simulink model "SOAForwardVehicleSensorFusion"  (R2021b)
settings: Solver=FixedStepAuto  StartTime=0.0  StopTime=scenario.StopTime  RelTol=1e-3

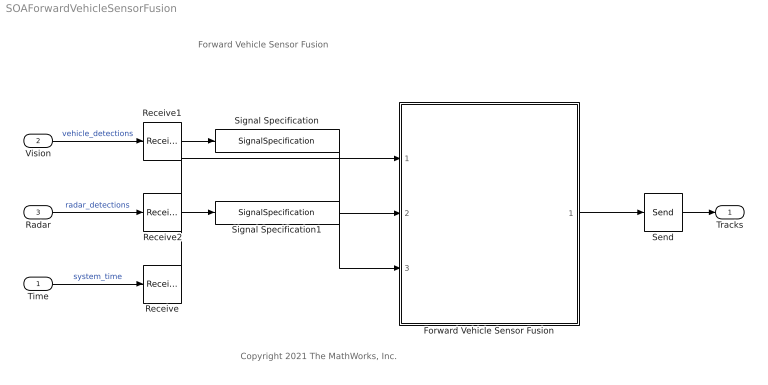
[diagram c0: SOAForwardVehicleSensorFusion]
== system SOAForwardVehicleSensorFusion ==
  note: Forward Vehicle Sensor Fusion
  note: Copyright 2021 The MathWorks, Inc.
  Time : Inport  OutputPortMessageModes=m  OutDataTypeStr=double  PortDimensions=[1 1]  SampleTime=[0.10000000000000001,0]
  Vision : Inport  Port=2  OutDataTypeStr=Bus: BusVision  PortDimensions=[1 1]  SampleTime=[0.10000000000000001,0]
  Radar : Inport  OutputPortMessageModes=m  Port=3  OutDataTypeStr=Bus: BusRadar  PortDimensions=[1 1]  SampleTime=[0.10000000000000001,0]
  Forward Vehicle Sensor Fusion : ModelReference  ModelNameDialog=ForwardVehicleSensorFusion.slx  SimulationMode=Normal  ModelReferenceVersion=4.3
  Receive : Receive  InputPortMessageModes=m  UseInternalQueue=off
  Receive1 : Receive  InputPortMessageModes=m  UseInternalQueue=off
  Receive2 : Receive  InputPortMessageModes=m  UseInternalQueue=off
  Send : Send  OutputPortMessageModes=m
  Signal Specification : SignalSpecification  OutDataTypeStr=Bus: BusVision
  Signal Specification1 : SignalSpecification  OutDataTypeStr=Bus: BusRadar
  Tracks : Outport  InputPortMessageModes=m  OutDataTypeStr=Bus: BusTrackerJPDA  PortDimensions=[1 1]  SampleTime=[0.10000000000000001,0]  VectorParamsAs1DForOutWhenUnconnected=off
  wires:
  Radar/1 -> Receive2/1  "radar_detections"
  Time/1 -> Receive/1  "system_time"
  Vision/1 -> Receive1/1  "vehicle_detections"
  Send/1 -> Tracks/1
  Receive1/1 -> Signal Specification/1
  Receive2/1 -> Signal Specification1/1
  Signal Specification1/1 -> Forward Vehicle Sensor Fusion/3
  Receive/1 -> Forward Vehicle Sensor Fusion/1
  Forward Vehicle Sensor Fusion/1 -> Send/1
  Signal Specification/1 -> Forward Vehicle Sensor Fusion/2
